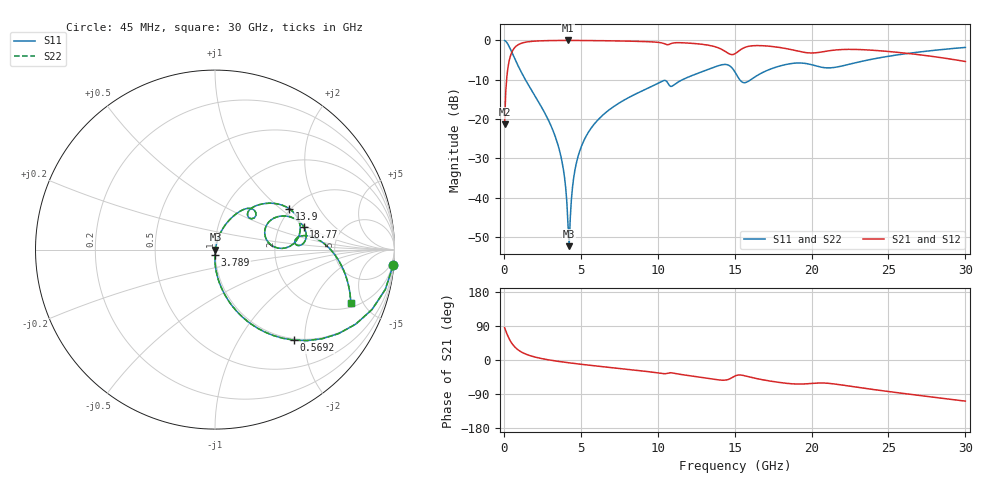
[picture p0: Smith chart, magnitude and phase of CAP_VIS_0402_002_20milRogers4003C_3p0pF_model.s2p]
! S-parameter model data by Modelithics Inc.  support@modelithics.com  813-866-6335  Tampa FL USA
! S-Parameter data specifications:
! Substrate: 20-mil Rogers 4003C, substrate thickness, H=0.508mm, Dielectric constant, Er=3.75
! PCB Mounting Pad Footprint: Pad width, PadW=0.50mm , Pad length, PadL=0.50mm , Pad gap, PadG (edge-to-edge)=0.40mm , Reference planes=1.4mm apart
! Created Wed Nov 18 12:46:09 2015
# hz S ma R 50
! 2 Port Network Data from SP1.SP block
! freq  magS11  angS11  magS21  angS21  magS12  angS12  magS22  angS22
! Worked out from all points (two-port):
!   401 points, 45 MHz to 30 GHz, reference 50 ohm
!   highest |S21| = -0.02 dB at 4.164 GHz (marker M1); lowest = -21.3 dB at 45 MHz (marker M2)
!   |S21| within 3 dB of the highest: 515.4 MHz to 14.47 GHz (13.96 GHz wide, 186 % of centre); 20.55 GHz to 25.53 GHz (4.976 GHz wide, 21.6 % of centre)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
!   lowest |S11| = -52.4 dB at 4.239 GHz (marker M3), VSWR 1.00, Z = 50.2 + j0.02 ohm
!   |S11| at or under -10 dB: 1.396 GHz to 11.61 GHz (10.21 GHz wide, 157 % of centre); 15.33 GHz to 16.06 GHz (728 MHz wide, 4.64 % of centre)
!   |S22| runs from -52.4 to 0.0 dB; largest |S21 - S12| = 0
!   S11 on the Smith chart (normalised r, x): 45 MHz: 1, -23; 569.2 MHz: 0.97, -1.77; 3.789 GHz: 1.00, -0.06; 13.9 GHz: 1.97, +1.15; 18.77 GHz: 2.71, +0.94; 30 GHz: 2.27, -4.02
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4.5e7  0.9963 -5.0  0.08595 85.0  0.08595 85.0  0.9963 -5.0
2.696625e8  0.8875 -27.9  0.4606 62.1  0.4606 62.1  0.8875 -27.9
5.692125e8  0.6687 -49.0  0.7428 41.0  0.7428 41.0  0.6687 -49.0
9.4365e8  0.4651 -63.8  0.8842 26.1  0.8842 26.1  0.4651 -63.8
1.467862e9  0.2988 -74.9  0.953 14.8  0.953 14.8  0.2988 -74.9
3.0405e9  0.08356 -89.2  0.9945 -0.5  0.9945 -0.5  0.08356 -89.2
3.789375e9  0.02776 -90.5  0.9973 -5.1  0.9973 -5.1  0.02776 -90.5
4.163812e9  0.004615 -66.8  0.9975 -7.1  0.9975 -7.1  0.004615 -66.8
4.2387e9  0.002404 4.7  0.9975 -7.5  0.9975 -7.5  0.002404 4.7
4.613138e9  0.02213 74.2  0.9971 -9.3  0.9971 -9.3  0.02213 74.2
5.062462e9  0.04608 75.2  0.9962 -11.5  0.9962 -11.5  0.04608 75.2
6.709988e9  0.1246 69.6  0.9888 -18.9  0.9888 -18.9  0.1246 69.6
1.007992e10  0.2887 52.4  0.941 -34.4  0.941 -34.4  0.2887 52.4
1.097858e10  0.2648 46.8  0.9245 -34.4  0.9245 -34.4  0.2648 46.8
1.389919e10  0.4729 28.7  0.8088 -52.2  0.8088 -52.2  0.4729 28.7
1.50225e10  0.395 1.4  0.6756 -42.2  0.6756 -42.2  0.395 1.4
1.569649e10  0.2903 17.0  0.8184 -42.0  0.8184 -42.0  0.2903 17.0
1.696958e10  0.4029 27.4  0.8513 -53.3  0.8513 -53.3  0.4029 27.4
1.876688e10  0.5097 14.6  0.7563 -62.9  0.7563 -62.9  0.5097 14.6
2.003996e10  0.4877 3.5  0.6909 -61.6  0.6909 -61.6  0.4877 3.5
2.505742e10  0.6302 1.3  0.7204 -83.5  0.7204 -83.5  0.6302 1.3
3e10  0.8137 -21.6  0.5381 -108.6  0.5381 -108.6  0.8137 -21.6
